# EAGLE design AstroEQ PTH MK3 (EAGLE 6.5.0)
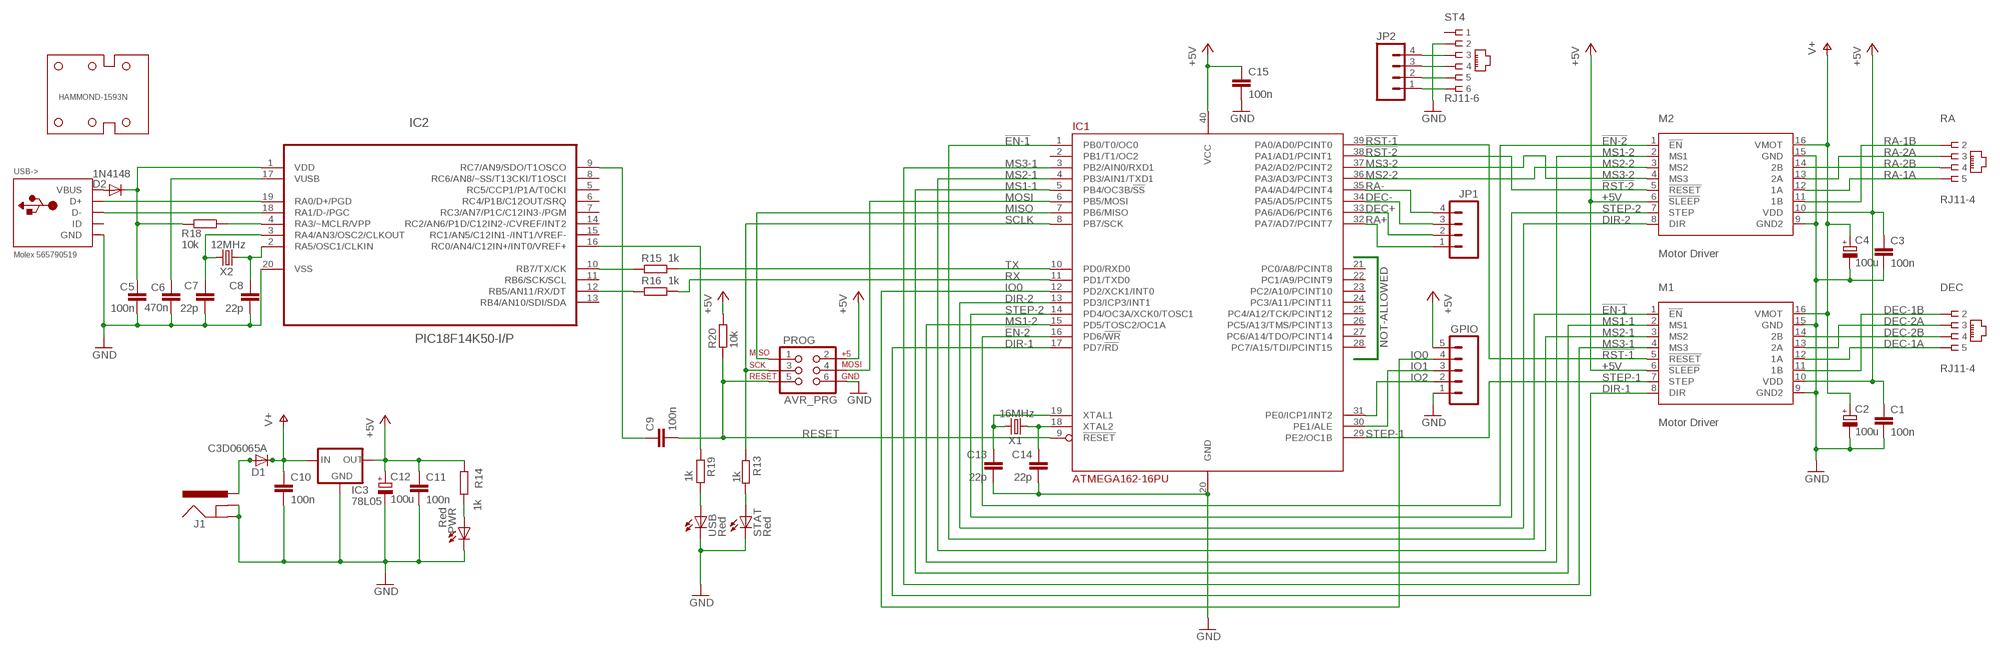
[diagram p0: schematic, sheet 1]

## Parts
C1  100n  C-EU025-024X044  [C025-024X044]
C2  100u  CPOL-EUE2.5-7  [E2,5-7]
C3  100n  C-EU025-024X044  [C025-024X044]
C4  100u  CPOL-EUE2.5-7  [E2,5-7]
C5  100n  C-EU025-024X044  [C025-024X044]
C6  470n  C-EU025-024X044  [C025-024X044]
C7  22p  C-EU025-024X044  [C025-024X044]
C8  22p  C-EU025-024X044  [C025-024X044]
C9  100n  C-EU025-024X044  [C025-024X044]
C10  100n  C-EU025-024X044  [C025-024X044]
C11  100n  C-EU025-024X044  [C025-024X044]
C12  100u  CPOL-EUE2.5-7  [E2,5-7]
C13  22p  C-EU025-024X044  [C025-024X044]
C14  22p  C-EU025-024X044  [C025-024X044]
C15  100n  C-EU025-024X044  [C025-024X044]
D1  C3D06065A  MUR820  [C221B1A]
D2  1N4148  DIODE1N4148  [DIODE-1N4148]
DEC  RJ11-4  [RJ11-NO_SHIELD-4]
GPIO  M05PTH  [1X05]
HAMMOND-1593N  HAMMOND-1593N  [HAMMOND-1593N]
IC1  ATMEGA162-16PU  [DIL40]
IC2  PIC18F14K50-I/P  [DIL20]
IC3  78L05  V_REG_78XXTO-92  [TO-92]
J1  POWER_JACKPTH  [POWER_JACK_PTH]
JP1  M04PTH  [1X04]
JP2  M04PTH  [1X04]
M1  Motor Driver  A4983CARRIER  [DIP16-W]
M2  Motor Driver  A4983CARRIER  [DIP16-W]
PROG  AVR_PRG  AVR_SPI_PRG_6PTH  [2X3]
PWR  Red  LED3MM  [LED3MM]
R13  1k  R-EU_0204/7  [0204/7]
R14  1k  R-EU_0204/7  [0204/7]
R15  1k  R-EU_0204/7  [0204/7]
R16  1k  R-EU_0204/7  [0204/7]
R18  10k  R-EU_0204/7  [0204/7]
R19  1k  R-EU_0204/7  [0204/7]
R20  10k  R-EU_0204/7  [0204/7]
RA  RJ11-4  [RJ11-NO_SHIELD-4]
ST4  RJ11-6  RJ11-2L-B  [RJ11-NO_SHIELD]
STAT  Red  LED3MM  [LED3MM]
USB  Red  LED3MM  [LED3MM]
USB->  Molex 565790519  USBMOLEX  [USB-MINIB-THM-MOLEX]
X1  16MHz  CRYSTALHC49US  [HC49US]
X2  12MHz  CRYSTALHC49US  [HC49US]

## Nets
!EN-1: IC1.1(PB0/T0/OC0) M1.1(!EN)
!EN-2: IC1.16(PD6/!WR) M2.1(!EN)
!RST-1: IC1.39(PA0/AD0/PCINT0) M1.5(!RESET)
!RST-2: IC1.38(PA1/AD1/PCINT1) M2.5(!RESET)
+5V: C1.1 C3.1 C11.1 C12.+ C15.1 GPIO.5 IC1.40(VCC) IC3.1(OUT) M1.6(!SLEEP) M1.10(VDD) M2.6(!SLEEP) M2.10(VDD) PROG.2 R14.1 R20.2
AVROSC1: C13.1 IC1.19(XTAL1) X1.2
AVROSC2: C14.1 IC1.18(XTAL2) X1.1
D+: IC2.19(RA0/D+/PGD) USB->.D+
D-: IC2.18(RA1/D-/PGC) USB->.D-
DEC+: IC1.33(PA6/AD6/PCINT6) JP1.2
DEC+B: JP2.2 ST4.5
DEC-: IC1.34(PA5/AD5/PCINT5) JP1.3
DEC-1A: DEC.5 M1.12(1A)
DEC-1B: DEC.2 M1.11(1B)
DEC-2A: DEC.3 M1.13(2A)
DEC-2B: DEC.4 M1.14(2B)
DEC-B: JP2.3 ST4.4
DIR-1: IC1.17(PD7/!RD) M1.8(DIR)
DIR-2: IC1.13(PD3/ICP3/INT1) M2.8(DIR)
DTR: C9.1 IC2.9(RC7/AN9/SDO/T1OSCO)
GND: C1.2 C2.- C3.2 C4.- C5.2 C6.1 C7.2 C8.2 C10.2 C11.2 C12.- C13.2 C14.2 C15.2 GPIO.1 IC1.20(GND) IC2.20(VSS) IC3.2(GND) J1.GND J1.GNDBREAK M1.9(GND2) M1.15(GND) M2.9(GND2) M2.15(GND) PROG.6 PWR.K(C) ST4.2 STAT.K(C) USB->.GND USB->.GND1(GND) USB->.GND4(GND) USB.K(C)
IO0: GPIO.4 IC1.12(PD2/XCK1/INT0)
IO1: GPIO.3 IC1.30(PE1/ALE)
IO2: GPIO.2 IC1.31(PE0/ICP1/INT2)
MCLR: IC2.4(RA3/~MCLR/VPP) R18.1
MISO: IC1.7(PB6/MISO) PROG.1
MOSI: IC1.6(PB5/MOSI) PROG.4
MS1-1: IC1.5(PB4/OC3B/!SS) M1.2(MS1)
MS1-2: IC1.15(PD5/TOSC2/OC1A) M2.2(MS1)
MS2-1: IC1.4(PB3/AIN1/TXD1) M1.3(MS2)
MS2-2: IC1.36(PA3/AD3/PCINT3) M2.3(MS2)
MS3-1: IC1.3(PB2/AIN0/RXD1) M1.4(MS3)
MS3-2: IC1.37(PA2/AD2/PCINT2) M2.4(MS3)
PWRLED: PWR.A R14.2
RA+: IC1.32(PA7/AD7/PCINT7) JP1.1
RA+B: JP2.1 ST4.6
RA-: IC1.35(PA4/AD4/PCINT4) JP1.4
RA-1A: M2.12(1A) RA.5
RA-1B: M2.11(1B) RA.2
RA-2A: M2.13(2A) RA.3
RA-2B: M2.14(2B) RA.4
RA-B: JP2.4 ST4.3
RESET: C9.2 IC1.9(!RESET) PROG.5 R20.1
RX: IC1.11(PD1/TXD0) R16.1
RX(USB): IC2.12(RB5/AN11/RX/DT) R16.2
SCLK: IC1.8(PB7/SCK) PROG.3 R13.1
STATLED: R13.2 STAT.A
STEP-1: IC1.29(PE2/OC1B) M1.7(STEP)
STEP-2: IC1.14(PD4/OC3A/XCK0/TOSC1) M2.7(STEP)
TX: IC1.10(PD0/RXD0) R15.1
TX(USB): IC2.10(RB7/TX/CK) R15.2
USBLED: R19.1 USB.A
USBOSC1: C8.1 IC2.2(RA5/OSC1/CLKIN) X2.1
USBOSC2: C7.1 IC2.3(RA4/AN3/OSC2/CLKOUT) X2.2
USBSTAT: IC2.16(RC0/AN4/C12IN+/INT0/VREF+) R19.2
V+: C2.+ C4.+ C10.1 D1.C IC3.3(IN) M1.16(VMOT) M2.16(VMOT)
VBUS: D2.A USB->.VBUS
VIN: D1.A J1.PWR
VPIC: C5.1 D2.C IC2.1(VDD) R18.2
VUSB: C6.2 IC2.17(VUSB)
Unconnected: IC1.2(PB1/T1/OC2) IC1.21(PC0/A8/PCINT8) IC1.22(PC1/A9/PCINT9) IC1.23(PC2/A10/PCINT10) IC1.24(PC3/A11/PCINT11) IC1.25(PC4/A12/TCK/PCINT12) IC1.26(PC5/A13/TMS/PCINT13) IC1.27(PC6/A14/TDO/PCINT14) IC1.28(PC7/A15/TDI/PCINT15) IC2.5(RC5/CCP1/P1A/T0CKI) IC2.6(RC4/P1B/C12OUT/SRQ) IC2.7(RC3/AN7/P1C/C12IN3-/PGM) IC2.8(RC6/AN8/~SS/T13CKI/T1OSCI) IC2.11(RB6/SCK/SCL) IC2.13(RB4/AN10/SDI/SDA) IC2.14(RC2/AN6/P1D/C12IN2-/CVREF/INT2) IC2.15(RC1/AN5/C12IN1-/INT1/VREF-) ST4.1 USB->.ID

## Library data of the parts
C1 C3 C5 C9-C11 C15 = resistor:C-EU: CAPACITOR, European symbol; MF: AVX; MPN: SR205C104KAR; OC_FARNELL: 1100367
C2 C4 C12 = resistor:CPOL-EU: POLARIZED CAPACITOR, European symbol; MF: MULTICOMP; MPN: MCGPR25V107M6.3X11; OC_FARNELL: 9451188
C6 = resistor:C-EU: CAPACITOR, European symbol; MF: KEMET; MPN: C320C474M5U5TA; OC_FARNELL: 1457660
C7 C8 C13 C14 = resistor:C-EU: CAPACITOR, European symbol; MF: AVX; MPN: SR151A220JAR; OC_FARNELL: 1100369
D1 = diode:MUR820: DIODE; MF: CREE; MPN: C3D06065A; OC_FARNELL: 1864928
D2 = SparkFun:DIODE: Diode; MF: MULTICOMP; MPN: 1N4148.; OC_FARNELL: 9565124
DEC RA = con-tycoelectronics:RJ11-4; MF: MOLEX; MPN: 95501-2641; OC_FARNELL: 1560166
GPIO = SparkFun:M05: Header 5 Standard 5-pin 0.1" header. Use with straight break away headers (SKU : PRT-00116), right angle break away headers (PRT-00553), swiss pins (PRT-00743), machine pins (PRT-00117), and female headers (PRT-00115). Molex polarized connector foot print use with SKU : PRT-08230 with associated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
HAMMOND-1593N = holes:HAMMOND-1593N; MF: HAMMOND; MPN: 1593NBK; OC_FARNELL: 9287566
IC1 = atmel:ATMEGA162: 8-bit RISC MICROCONTROLLER 16K Bytes internal flash program memory 1K Bytes internal SRAM Upto 64K Bytes optional external memory space 512 Bytes EEPROM Two 8-bit timers Two 16-bit timers Dual programmable serial USARTs Master/Slave serial SPI interface Source: ATMEGA162_DIP40.lbr; MF: ATMEL; MPN: ATMEGA162-16PU; OC_FARNELL: 9171169
IC2 = microchip:PIC18F14K50-I/P: USB Flash Microcontrollers; MF: MICROCHIP; MPN: PIC18F14K50-I/P; OC_FARNELL: 1648501; OC_NEWARK: 77M3103; PACKAGE: DIP-20; SUPPLIER: Microchip
IC3 = SparkFun:V_REG_78XX: Voltage Regulator Standard 7805 5V regulator. IGO (Input Ground Output). Spark Fun Electronics SKU : COM-00107; MF: FAIRCHILD SEMICONDUCTOR; MPN: LM78L05ACZX; OC_FARNELL: 1467367
J1 = SparkFun:POWER_JACK: Power Jack This is the standard 5.5mm barrel jack for power. The PTH is the most common, proven, reliable, footprint. All others are experimental. The Slot footprint only works if the mill layer is transmitted to the PCB fab house so be warned. Spark Fun Electronics SKU : PRT-00119. Mating wall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; MF: MULTICOMP; MPN: MJ-179PH; OC_FARNELL: 1737246
JP1 JP2 = SparkFun:M04: Header 4 Standard 4-pin 0.1" header. Use with straight break away headers (SKU : PRT-00116), right angle break away headers (PRT-00553), swiss pins (PRT-00743), machine pins (PRT-00117), and female headers (PRT-00115). Molex polarized connector foot print use with SKU : PRT-08231 with associated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
M1 M2 = A4983Carrier:A4983CARRIER; MF: SAMTEC; MPN: CES-116-01-T-S; OC_FARNELL: 1667522
PROG = SparkFun:AVR_SPI_PRG_6: AVR ISP 6 Pin This is the reduced ISP connector for AVR programming. Common on Arduino. This footprint will take up less PCB space and can be used with a 10-pin to 6-pin adapter such as SKU: BOB-08508; MF: TE CONNECTIVITY / AMP; MPN: 826632-3; OC_FARNELL: 3418492
PWR STAT USB = led:LED: LED; MF: KINGBRIGHT; MPN: L-424HDT; OC_FARNELL: 1142499
R13-R16 R19 = rcl:R-EU_: RESISTOR, European symbol; MF: MULTICOMP; MPN: MF12 1K; OC_FARNELL: 9342400
R18 R20 = rcl:R-EU_: RESISTOR, European symbol; MF: MULTICOMP; MPN: MF12 10K; OC_FARNELL: 9342419
ST4 = con-tycoelectronics:RJ11: CORCOM Modular RJ Jacks No Shield Source: www.tycoelectronics.com .. ENG_DS_1654001_1099_RJ_L_0507.pdf; MF: TYCO ELECTRONICS; MPN: RJ11-2L-B; OC_FARNELL: unknown; OC_NEWARK: 83F4463
USB-> = adafruit:USB: USB Connectors USBMINIB - Surface Mount Female Mini-B USB Connector 4UConnector: 06564 By microbuilder.eu Thru-hole RA Female Mini-B USB Connector 4UConnector: 18732 By ladyada.net; MF: MOLEX; MPN: 565790519; OC_FARNELL: 1125347
X1 = SparkFun:CRYSTAL: Crystals; MF: TXC; MPN: 9B-16.000MEEJ-B; OC_FARNELL: 1842217
X2 = SparkFun:CRYSTAL: Crystals; MF: TXC; MPN: 9B-12.000MAAJ-B; OC_FARNELL: 1842203

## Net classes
1 power: width 0.61 mm, drill 0.711 mm, clearance 0.203 mm
2 gnd: width 0.305 mm, drill 0.711 mm, clearance 0.203 mm
3 usbvcc: width 0.508 mm, drill 0.711 mm, clearance 0.203 mm

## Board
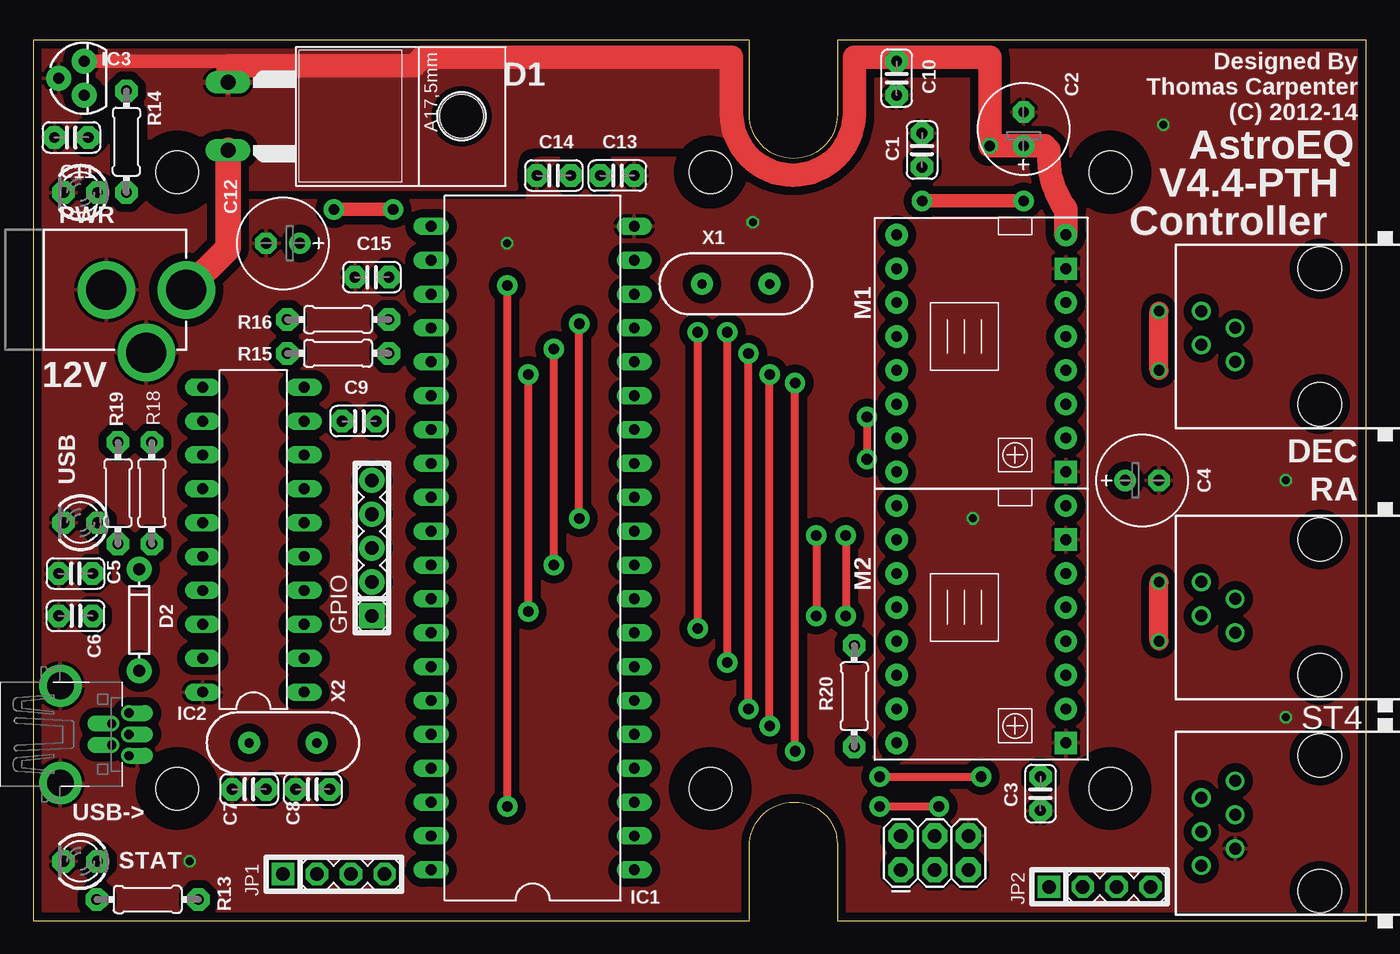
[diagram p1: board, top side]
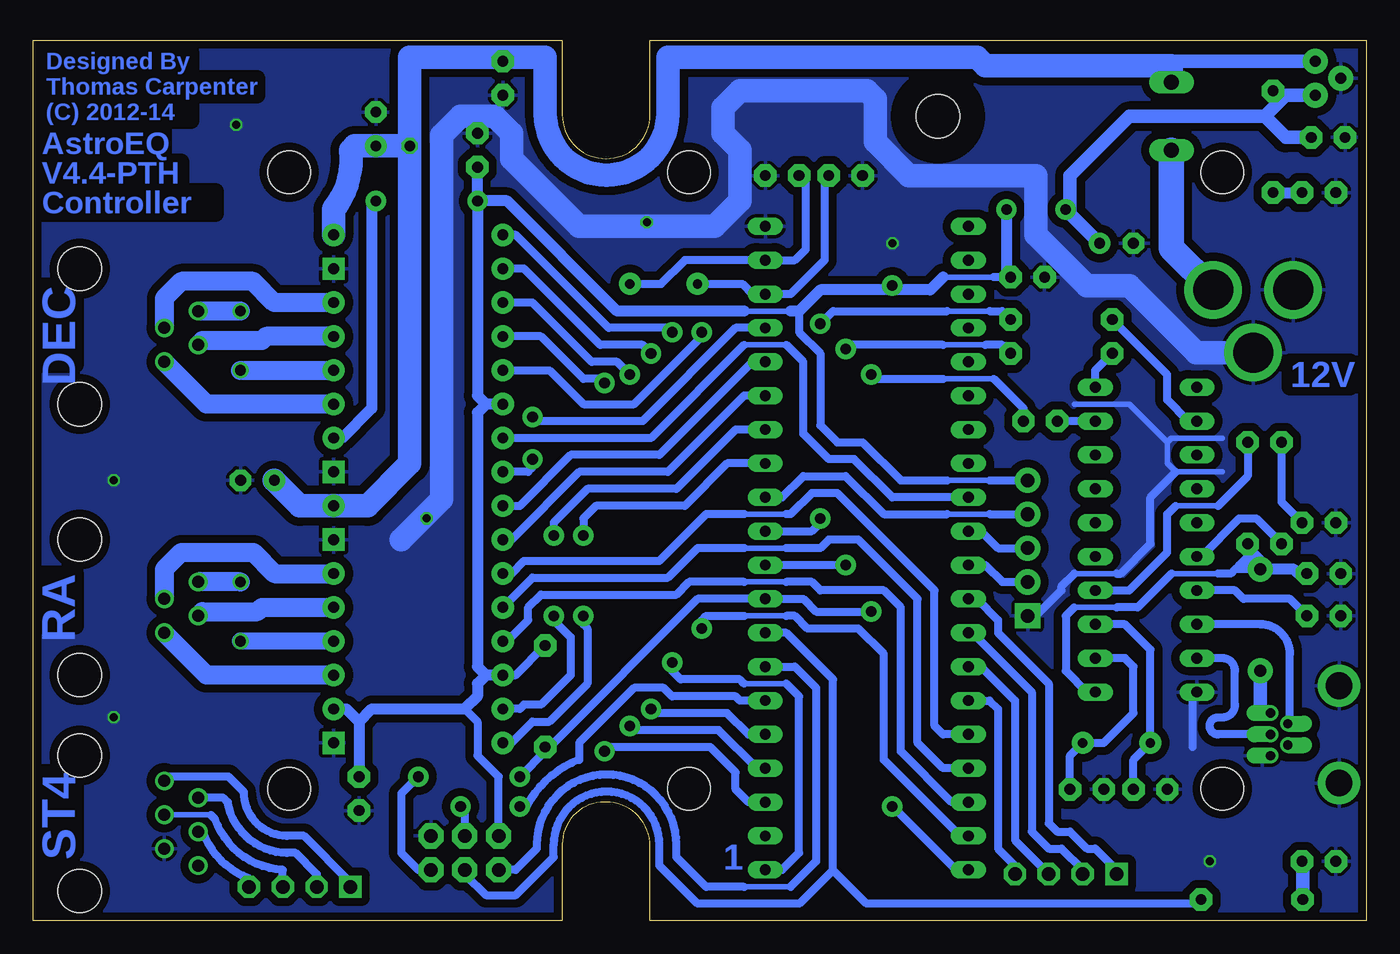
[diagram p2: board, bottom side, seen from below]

Size 100 x 66.04 mm. Coordinates in mm from the lower left corner, seen from the top.
Outline: 57.02,8.89 57.15,8.89
Copper layers (1*16): Top 0.035mm / dielectric 1.5mm / Bottom 0.035mm
Design rules "default *": minimum track width 6mil, minimum drill 12mil, track to track 6mil, track to pad 6mil, pad to pad 6mil, via to via 6mil, smd to smd 0mil, copper to edge 10mil, drill to drill 10mil, minimum pad ring 10mil, minimum via ring 6mil, stop-mask expansion 2mil, vias tented up to drill 1mm, thermal gap 10mil
tKeepout: area 78.3,7.4 to 83.3,12.4; area 78.3,53.6 to 83.3,58.6; area 48.3,7.4 to 53.3,12.4; area 8.3,7.4 to 13.3,12.4; area 48.3,53.6 to 53.3,58.6; area 8.3,53.6 to 13.3,58.6
bKeepout: area 78.3,7.4 to 83.3,12.4; area 78.3,53.6 to 83.3,58.6; area 48.3,7.4 to 53.3,12.4; area 8.3,7.4 to 13.3,12.4; area 48.3,53.6 to 53.3,58.6; area 8.3,53.6 to 13.3,58.6
tRestrict: area 78.3,53.6 to 83.3,58.6; area 78.3,7.4 to 83.3,12.4; area 48.3,7.4 to 53.3,12.4; area 8.3,7.4 to 13.3,12.4; area 8.3,53.6 to 13.3,58.6; area 6.3,56.2 to 7.9,60.6; 1 lines

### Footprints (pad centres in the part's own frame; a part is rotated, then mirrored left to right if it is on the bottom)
C025-024X044 = drill 0.813 pad 1.676 octagon: 1 -1.27,0; 2 1.27,0
E2,5-7 = drill 0.813 pad 1.6: + -1.27,0 | drill 0.813 pad 1.6 octagon: - 1.27,0
C221B1A = drill 1.118 long: A 2.54,-6.35; C -2.54,-6.35 | hole 3.302: 0,11.176
DIODE-1N4148 = drill 0.9 pad 1.88: A -3.81,0; C 3.81,0
RJ11-NO_SHIELD-4 = drill 0.9 pad 1.4: 2 -1.905,6.35; 3 -0.635,8.89; 4 0.635,6.35; 5 1.905,8.89 | hole 3.251: -5.08,0; 5.08,0
1X05 = drill 1.016 pad 1.88 square: 1 0,0 | drill 1.016 pad 1.88: 2 2.54,0; 3 5.08,0; 4 7.62,0; 5 10.16,0
HAMMOND-1593N = hole 3.2: 10.795,9.906; 10.795,56.134; 50.8,9.906; 50.8,56.134; 80.797,9.906; 80.797,56.134
DIL40 = drill 0.813 long: 1 -24.13,-7.62; 2 -21.59,-7.62; 3 -19.05,-7.62; 4 -16.51,-7.62; 5 -13.97,-7.62; 6 -11.43,-7.62; 7 -8.89,-7.62; 8 -6.35,-7.62; 9 -3.81,-7.62; 10 -1.27,-7.62; 11 1.27,-7.62; 12 3.81,-7.62; 13 6.35,-7.62; 14 8.89,-7.62; 15 11.43,-7.62; 16 13.97,-7.62; 17 16.51,-7.62; 18 19.05,-7.62; 19 21.59,-7.62; 20 24.13,-7.62; 21 24.13,7.62; 22 21.59,7.62; 23 19.05,7.62; 24 16.51,7.62; 25 13.97,7.62; 26 11.43,7.62; 27 8.89,7.62; 28 6.35,7.62; 29 3.81,7.62; 30 1.27,7.62; 31 -1.27,7.62; 32 -3.81,7.62; 33 -6.35,7.62; 34 -8.89,7.62; 35 -11.43,7.62; 36 -13.97,7.62; 37 -16.51,7.62; 38 -19.05,7.62; 39 -21.59,7.62; 40 -24.13,7.62
DIL20 = drill 0.813 long: 1 -3.81,11.43; 2 -3.81,8.89; 3 -3.81,6.35; 4 -3.81,3.81; 5 -3.81,1.27; 6 -3.81,-1.27; 7 -3.81,-3.81; 8 -3.81,-6.35; 9 -3.81,-8.89; 10 -3.81,-11.43; 11 3.81,-11.43; 12 3.81,-8.89; 13 3.81,-6.35; 14 3.81,-3.81; 15 3.81,-1.27; 16 3.81,1.27; 17 3.81,3.81; 18 3.81,6.35; 19 3.81,8.89; 20 3.81,11.43
TO-92 = drill 0.813 pad 1.88: 1 -1.27,0; 2 0,1.905; 3 1.27,0
POWER_JACK_PTH = drill 2.997 pad 4.318: GND 0,7.7; GNDBREAK 4.7,10.7; PWR 0,13.7
1X04 = drill 1.016 pad 1.676 square: 1 0,0 | drill 1.016 pad 1.676 octagon: 2 2.54,0; 3 5.08,0; 4 7.62,0
DIP16-W = drill 0.813 pad 1.676: 1 -8.89,-6.35; 2 -6.35,-6.35; 3 -3.81,-6.35; 4 -1.27,-6.35; 5 1.27,-6.35; 6 3.81,-6.35; 7 6.35,-6.35; 8 8.89,-6.35; 10 6.35,6.35; 11 3.81,6.35; 12 1.27,6.35; 13 -1.27,6.35; 14 -3.81,6.35; 16 -8.89,6.35 | drill 0.813 pad 1.676 square: 9 8.89,6.35; 15 -6.35,6.35
2X3 = drill 1.016 pad 1.88 octagon: 1 0,0; 2 0,2.54; 3 2.54,0; 4 2.54,2.54; 5 5.08,0; 6 5.08,2.54
LED3MM = drill 0.813 pad 1.676 octagon: A -1.27,0; K 1.27,0
0204/7 = drill 0.813 pad 1.676 octagon: 1 -3.81,0; 2 3.81,0
RJ11-NO_SHIELD = drill 0.9 pad 1.4: 1 -3.175,8.89; 2 -1.905,6.35; 3 -0.635,8.89; 4 0.635,6.35; 5 1.905,8.89; 6 3.175,6.35 | hole 3.251: -5.08,0; 5.08,0
USB-MINIB-THM-MOLEX = drill 0.7 offset: D+ 0,9.72; D- -0.8,8.42; GND 1.6,9.72; ID 0.8,8.42; VBUS -1.6,9.72 | drill 2 pad 3.175: GND1 -3.65,4.57; GND4 3.65,4.57
HC49US = drill 0.7 pad 1.651: 1 -2.54,0; 2 2.54,0

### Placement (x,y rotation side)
C1  66.67,57.78 90 top
C2  74.3,59.37 90 top
C3  75.56,9.53 270 top
C4  83.19,33.02 0 top
C5  3.17,26.04 180 top
C6  3.17,22.86 0 top
C7  16.19,9.84 180 top
C8  20.95,9.84 180 top
C9  24.45,37.47 0 top
C10  64.77,63.18 270 top
C11  2.86,58.74 180 top
C12  18.73,50.8 180 top
C13  43.81,55.88 0 top
C14  39.05,55.88 180 top
C15  25.4,48.26 180 top
D1  20.95,60.33 270 top
D2  7.94,22.54 90 top
DEC  96.52,43.81 90 top
GPIO  25.4,22.86 90 top
HAMMOND-1593N  0,0 0 top
IC1  37.47,27.94 90 top
IC2  16.51,28.57 180 top
IC3  3.81,63.18 90 top
J1  -2.22,47.31 270 top
JP1  18.73,3.49 0 top
JP2  76.2,2.54 0 top
M1  71.12,42.55 270 top
M2  71.12,22.23 270 top
PROG  65.09,3.81 0 top
PWR  3.54,54.61 180 top
R13  8.57,1.59 180 top
R14  6.99,58.42 270 top
R15  22.86,42.55 180 top
R16  22.86,45.09 180 top
R18  8.89,32.07 270 top
R19  6.35,32.07 270 top
R20  61.59,16.83 90 top
RA  96.52,23.5 90 top
ST4  96.52,7.3 90 top
STAT  3.54,4.45 180 top
USB  3.54,29.84 180 top
USB->  -2.54,13.97 270 top
X1  52.7,47.75 0 top
X2  18.73,13.34 180 top

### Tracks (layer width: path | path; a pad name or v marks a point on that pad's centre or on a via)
!EN-1  (via drill 0.8 pad 1.52)
  Top 0.61: v52.07,19.37 v52.07,44.13
  Bottom 0.406: 43.5,17.78 46.67,17.78
  Bottom 0.61: IC1.1 43.81,3.81 42.55,5.08 42.55,16.83 43.5,17.78 | 46.67,17.78 46.99,18.1 51.44,18.1 52.07,18.73 v52.07,19.37 | v52.07,44.13 52.39,44.45 56.83,44.45 63.82,51.44 M1.1
!EN-2
  Bottom 0.61: IC1.16 46.04,41.91 53.02,34.92 59.69,34.92 63.5,31.11 M2.1
!RST-1  (via drill 0.8 pad 1.52)
  Top 0.61: v49.85,44.13 v49.85,21.91
  Bottom 0.406: 43.5,22.86 46.67,22.86
  Bottom 0.61: IC1.39 30.48,6.35 36.2,12.06 36.2,20 38.1,21.91 41.91,21.91 42.86,22.86 43.5,22.86 | M1.5 61.28,41.27 58.74,38.73 54.93,38.73 49.85,43.81 v49.85,44.13 | v49.85,21.91 49.85,22.54 49.53,22.86 46.67,22.86
!RST-2
  Bottom 0.406: 43.5,25.4 46.67,25.4
  Bottom 0.61: IC1.38 31.11,8.89 34.92,12.7 34.92,23.5 36.2,24.77 40.96,24.77 41.59,25.4 43.5,25.4 | 46.67,25.4 50.8,25.4 51.75,24.45 61.91,24.45 62.87,23.5 62.87,22.54 64.45,20.95 M2.5
+5V  (via drill 0.8 pad 1.52)
  Top 0.61: v35.56,47.62 v35.56,8.57
  Top 1.016: v66.67,53.98 v74.3,53.98 | v22.54,53.34 v26.99,53.34
  Bottom 0.406: 27.94,48.26 31.75,48.26 | 43.18,45.72 46.67,45.72 | 31.43,33.02 28.26,33.02
  Bottom 0.61: 26.99,48.26 27.94,48.26 | PROG.2 65.09,10.79 66.67,12.38 66.67,14.92 67.63,15.88 | v35.56,47.62 35.56,47.31 | IC1.40 30.8,3.81 v35.56,8.57 | M2.6 63.82,18.41 R20.2 | 42.55,45.72 42.55,44.13 40.96,42.55 40.96,37.15 39.69,35.88 37.78,35.88 34.92,33.02 31.43,33.02 | 28.26,33.02 GPIO.5
  Bottom 0.813: v66.67,53.98 C1.1 | C15.1 26.99,48.26 v26.99,53.34 | 31.75,48.26 32.7,47.31 35.56,47.31 40.96,47.31 42.55,45.72 43.18,45.72 | 46.67,45.72 56.2,45.72 64.45,53.98 v66.67,53.98 | 22.23,53.66 22.23,53.34 v22.54,53.34 | v66.67,53.98 66.67,39.37 66.04,38.73 | 66.04,38.73 66.67,38.1 66.67,19.05 66.04,18.41 | 66.04,18.41 66.67,17.78 66.67,16.83 67.63,15.88 74.61,15.88 75.56,14.92 | M2.6 66.04,18.41 | M1.6 66.04,38.73 | v74.3,53.98 74.61,53.66 74.61,38.42 76.83,36.2 M1.10 | 75.56,14.92 C3.1 | M2.10 76.52,15.88 75.56,14.92
  Bottom 1.016: IC3.1 6.03,61.91 6.35,61.59 | 6.35,61.59 7.62,60.33 | 7.62,60.33 17.78,60.33 22.23,55.88 22.23,53.66 22.23,53.02 C12.+ | R14.1 6.35,61.59 | C11.1 6.03,58.74 7.62,60.33
AVROSC1
  Bottom 0.61: C13.1 42.07,55.4 42.07,50.32 42.86,49.53 IC1.19 51.12,49.53 52.9,47.75 X1.2
AVROSC2
  Bottom 0.61: C14.1 40.64,55.56 40.64,49.53 43.18,46.99 IC1.18 46.04,46.99 46.8,47.75 X1.1
D+
  Bottom 0.61: USB->.D+ 11.11,13.97 arc90 11.75,14.61 arc90 11.11,15.24 10.79,15.24 arc-90 9.84,16.19 9.84,18.73 arc-90 10.79,19.68 IC2.19
D-
  Bottom 0.61: USB->.D- 5.71,14.77 5.71,20 arc-90 7.94,22.23 IC2.18
DEC+
  Bottom 0.61: IC1.33 29.53,21.59 25.08,17.14 25.08,6.67 23.81,5.4 22.86,5.4 21.27,3.81 JP1.2
DEC+B
  Bottom 0.61: JP2.2 78.74,3.49 80.33,5.08 80.96,5.08 arc80 85.41,8.89 85.72,9.21 ST4.5
DEC-
  Bottom 0.61: IC1.34 28.89,19.05 26.35,16.51 26.35,6.03 JP1.3
DEC-1A  (via drill 0.8)
  Top 1.422: v84.45,41.27 v84.45,45.72
  Bottom 1.422: v84.45,45.72 DEC.5 | v84.45,41.27 M1.12
DEC-1B
  Bottom 1.422: M1.11 87,38.73 DEC.2
DEC-2A
  Bottom 1.422: M1.13 82.55,43.81 82.87,43.5 87.31,43.5 DEC.3
DEC-2B
  Bottom 1.422: M1.14 81.92,46.35 83.5,47.94 88.9,47.94 90.17,46.67 DEC.4
DEC-B
  Bottom 0.406: 86.68,7.94 ST4.4
  Bottom 0.61: 86.68,7.94 86.36,7.62 arc-68 81.28,3.81 JP2.3
DIR-1  (via drill 0.8 pad 1.52)
  Top 0.61: v62.55,37.78 v62.55,34.61
  Bottom 0.61: IC1.17 47.31,44.45 54.29,37.47 62.23,37.47 v62.55,37.78 | v62.55,34.61 62.55,33.97 62.87,33.66 M1.8
DIR-2  (via drill 0.8 pad 1.52)
  Top 0.61: v58.74,28.89 v58.74,22.86
  Bottom 0.61: M2.8 64.14,13.34 62.55,14.92 61.28,14.92 58.42,17.78 58.42,21.91 58.74,22.23 v58.74,22.86 | IC1.13 47.94,34.29 51.12,31.11 57.78,31.11 58.74,30.16 v58.74,28.89
DTR
  Bottom 0.61: IC2.9 C9.1
GND  (via drill 0.6)
  Bottom 0.406: 21.91,26.04 18.73,26.04 | 10.79,33.66 14.29,33.66 14.92,34.29 14.92,35.88 | 14.92,35.88 14.61,36.2 10.79,36.2 | 14.92,35.88 17.78,38.73 21.91,38.73
  Bottom 0.61: 13.02,13.02 13.02,16.83 IC2.20 | GPIO.1 24.77,22.86 22.86,24.77 22.86,25.08 21.91,26.04 | 18.73,26.04 18.41,26.04 16.19,28.26 16.19,31.75 14.29,33.66
  Bottom 1.778: J1.GNDBREAK 12.76,42.61 17.78,47.62 20.95,47.62 24.77,51.44 24.77,55.88 34.29,55.88 36.83,58.42 36.83,61.59 37.47,62.23 46.99,62.23 48.26,60.96 48.26,59.05 46.99,57.78 46.99,53.98 48.9,52.07 59.05,52.07 64.14,57.15 64.14,59.05 65.41,60.33 67.94,60.33 69.37,58.9 69.37,31.59 72.39,28.57
  other vias: 35.56,50.8 93.98,15.24 84.77,59.69 93.98,33.02 70.48,30.16 53.98,52.39 11.75,4.45
  pour Top (isolate 0.61, rank 2): -1.27,66.99 101.03,66.99 101.03,-0.95 -1.27,-0.95
  pour Bottom (isolate 0.61): -1.27,66.99 101.03,66.99 101.03,-0.95 -1.27,-0.95
IO0
  Bottom 0.406: 31.43,30.48 28.26,30.48
  Bottom 0.61: IC1.12 43.81,31.75 42.23,33.34 39.05,33.34 36.2,30.48 31.43,30.48 | 28.26,30.48 GPIO.4
IO1
  Bottom 0.61: IC1.30 28.89,29.21 27.62,27.94 GPIO.3
IO2
  Bottom 0.61: IC1.31 28.57,26.67 27.3,25.4 GPIO.2
MCLR
  Bottom 0.406: 14.29,31.11 11.11,31.11
  Bottom 0.61: IC2.4 17.78,24.77 14.92,27.62 14.92,30.48 14.29,31.11 | 11.11,31.11 8.89,33.34 R18.1
MISO
  Bottom 0.406: 43.18,2.54 46.67,2.54
  Bottom 0.61: IC1.7 42.86,19.05 41.27,17.46 41.27,4.45 43.18,2.54 | 46.67,2.54 49.53,2.54 51.75,4.76 51.75,5.71 arc-180 62.23,5.71 62.23,5.4 63.82,3.81 PROG.1
MOSI  (via drill 0.8 pad 1.52)
  Top 0.61: v63.5,8.57 v67.94,8.57
  Bottom 0.61: IC1.6 46.99,16.51 47.31,16.83 52.07,16.83 52.7,17.46 54.93,17.46 59.05,13.34 59.05,12.06 arc-42 63.01,8.57 v63.5,8.57 | v67.94,8.57 67.63,8.26 PROG.4
MS1-1  (via drill 0.8 pad 1.52)
  Top 0.61: v53.66,15.88 v53.66,42.55
  Bottom 0.61: IC1.5 46.35,13.97 47.94,15.56 53.34,15.56 v53.66,15.88 | v53.66,42.55 54.29,43.18 57.47,43.18 63.18,48.9 M1.2
MS1-2
  Bottom 0.61: IC1.15 46.67,39.37 52.39,33.66 59.05,33.66 64.14,28.57 M2.2
MS2-1  (via drill 0.8 pad 1.52)
  Top 0.61: v55.24,14.61 v55.24,40.96
  Bottom 0.61: IC1.4 45.72,11.43 48.58,14.29 54.93,14.29 v55.24,14.61 | v55.24,40.96 56.2,41.91 58.1,41.91 62.55,46.35 M1.3
MS2-2
  Bottom 0.406: 43.5,30.48 46.67,30.48
  Bottom 0.61: IC1.36 31.75,13.97 32.38,14.61 32.38,24.77 39.69,32.07 41.59,32.07 43.18,30.48 43.5,30.48 | 46.67,30.48 49.53,30.48 53.02,26.99 63.18,26.99 64.14,26.04 M2.3
MS3-1  (via drill 0.8 pad 1.52)
  Top 0.61: v57.15,12.7 v57.15,40.32
  Bottom 0.61: IC1.3 46.35,8.89 47.31,9.84 47.31,11.11 49.21,13.02 56.83,13.02 v57.15,12.7 | v57.15,40.32 57.47,40.64 58.74,40.64 61.91,43.81 M1.4
MS3-2
  Bottom 0.406: 43.5,27.94 46.67,27.94
  Bottom 0.61: IC1.37 31.75,11.43 33.66,13.34 33.66,24.13 38.1,28.57 40.32,28.57 40.96,27.94 43.5,27.94 | 46.67,27.94 50.16,27.94 52.39,25.72 62.55,25.72 M2.4
PWRLED
  Bottom 0.813: R14.2 PWR.A
RA+
  Bottom 0.61: IC1.32 29.21,24.13 27.62,22.54 27.62,21.59 23.81,17.78 23.81,7.3 23.18,6.67 22.23,6.67 20.95,5.4 20.32,5.4 18.73,3.81 JP1.1
RA+B
  Bottom 0.61: JP2.1 76.2,2.86 79.69,6.35 80.96,6.35 arc90 84.2,9.65 85.34,10.79 89.85,10.79 ST4.6
RA-
  Bottom 0.61: IC1.35 28.26,16.51 27.62,15.88 27.62,5.4 26.35,4.13 JP1.4
RA-1A  (via drill 0.8)
  Top 1.422: v84.45,20.95 v84.45,25.4
  Bottom 1.27: M2.12 v84.45,20.95
  Bottom 1.422: v84.45,25.4 RA.5
RA-1B
  Bottom 1.422: M2.11 87,18.41 RA.2
RA-2A
  Bottom 1.422: RA.3 87.31,23.18 83.19,23.18 82.87,23.5 M2.13
RA-2B
  Bottom 1.422: M2.14 81.92,26.04 83.5,27.62 88.9,27.62 90.17,26.35 RA.4
RA-B
  Bottom 0.61: ST4.3 87.31,6.67 arc-48 83.82,3.17 JP2.4
RESET  (via drill 0.8 pad 1.52)
  Top 0.61: v63.5,10.79 v71.12,10.79 | v37.15,23.18 v37.15,40.96
  Bottom 0.406: 31.75,40.64 27.94,40.64
  Bottom 0.61: v63.5,10.79 61.59,12.7 R20.1 61.28,13.02 50.16,24.13 IC1.9 42.23,24.13 41.27,23.18 v37.15,23.18 | v71.12,10.79 72.39,9.53 72.39,5.08 71.12,3.81 PROG.5 | v37.15,40.96 36.83,40.64 31.75,40.64 | 27.94,40.64 25.72,38.42 C9.2
RX  (via drill 0.8 pad 1.52)
  Top 0.61: v40.96,30.16 v40.96,44.77
  Bottom 0.406: 31.43,45.72 28.26,45.72
  Bottom 0.61: 31.43,45.72 40.01,45.72 v40.96,44.77 | 28.26,45.72 27.3,45.72 R16.1 | IC1.11 41.59,29.21 40.96,29.84 v40.96,30.16
RX(USB)
  Bottom 0.61: IC2.12 13.34,37.47 14.92,39.05 14.92,40.96 R16.2
SCLK
  Bottom 0.61: R13.1 12.7,1.27 37.49,1.27 40.01,3.79 | 40.01,3.79 40.01,18.1 43.5,21.59 IC1.8 | 40.01,3.79 42.52,1.27 50.16,1.27 53.02,4.13 53.02,5.71 arc-180 60.96,5.71 60.96,4.76 63.82,1.91 66.04,1.91 67.63,3.49 PROG.3
STATLED
  Bottom 1.016: STAT.A 4.76,4.49 R13.2
STEP-1
  Bottom 0.406: 43.5,43.18 46.67,43.18
  Bottom 0.61: IC1.29 35.56,31.75 38.42,34.61 40.32,34.61 42.23,36.51 42.23,41.91 43.5,43.18 | 46.67,43.18 53.66,36.2 M1.7
STEP-2  (via drill 0.8 pad 1.52)
  Top 0.61: v60.96,28.89 v60.96,22.86
  Bottom 0.61: IC1.14 47.31,36.83 51.75,32.38 58.42,32.38 60.96,29.84 v60.96,28.89 | v60.96,22.86 60.96,22.54 59.69,21.27 59.69,18.41 61.91,16.19 63.18,16.19 63.5,15.88 M2.7
TX  (via drill 0.8 pad 1.52)
  Top 0.61: v39.05,26.67 v39.05,42.86
  Bottom 0.406: 28.57,43.18 31.75,43.18
  Bottom 0.61: v39.05,26.67 IC1.10 | R15.1 27.3,43.18 28.57,43.18 | 31.75,43.18 38.73,43.18 v39.05,42.86
TX(USB)
  Bottom 0.61: IC2.10 20.32,41.27 R15.2
USBLED
  Bottom 0.61: USB.A 6.35,31.39 R19.1
USBOSC1
  Bottom 0.61: IC2.2 18.1,19.68 17.46,19.05 17.46,15.56 19.68,13.34 X2.1 22.23,12.38 C8.1
USBOSC2
  Bottom 0.61: IC2.3 18.1,22.23 16.19,20.32 X2.2 17.46,12.06 C7.1
USBSTAT
  Bottom 0.61: IC2.16 12.38,27.3 9.53,30.16 8.26,30.16 R19.2
V+  (via drill 0.8)
  Top 1.016: IC3.3 14.61,64.45 14.61,63.82
  Top 1.778: 14.61,63.82 D1.C 14.61,64.14 28.57,64.14 29.21,64.77 52.39,64.77 52.39,60.52 arc180 61.59,60.52 61.59,64.77 71.75,64.77 v71.75,58.1 C2.+ 75.88,58.1 76.2,57.78 76.2,57.15 arc37 77.47,53.34 M1.16
  Bottom 0.61: C10.1 64.77,64.77 | D1.C 14.61,63.5 14.61,64.45 14.29,64.45
  Bottom 1.016: IC3.3 14.29,64.45
  Bottom 1.778: v71.75,58.1 71.75,64.77 64.77,64.77 61.59,64.77 61.59,60.52 arc-180 52.39,60.52 52.39,64.77 29.21,64.77 28.57,64.14 14.61,64.14 14.61,63.5 | v71.75,58.1 C2.+ 75.88,58.1 76.2,57.78 arc45 77.47,53.34 M1.16 | v71.75,58.1 71.75,34.29 74.93,31.11 M2.16 80.01,31.11 C4.+
  pour Top (isolate 0.61): 3.17,66.04 3.17,61.28 6.99,61.28 6.99,54.93 36.2,54.93 36.2,56.83 arc-90 37.47,58.1 50.8,58.1 50.8,57.47 57.15,57.47 57.15,66.04
VBUS
  Bottom 1.016: USB->.VBUS 7.94,15.57 D2.A
VIN
  Top 1.93: J1.PWR 14.61,50.44 D1.A
  Bottom 1.93: J1.PWR 14.61,50.44 D1.A
VPIC
  Bottom 0.406: 11.11,26.04 14.61,26.04 | 18.73,23.5 21.91,23.5
  Bottom 0.61: 14.61,26.04 17.14,23.5 18.73,23.5 | 21.91,23.5 22.54,22.86 22.54,18.73 20.95,17.14 IC2.1 | 11.11,26.04 10.16,26.04 9.84,26.35 | D2.C 9.84,26.35 | 9.84,26.35 9.53,26.67 | 8.57,27.62 9.53,26.67 | 9.53,26.67 8.89,26.67 8.26,27.3
  Bottom 0.813: C5.1 5.08,26.04 5.4,26.35 D2.C 7.94,26.99 8.57,27.62 8.89,27.94 R18.2
VUSB
  Bottom 0.61: C6.2 5.71,24.13 9.21,24.13 9.84,24.77 IC2.17

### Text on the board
Bottom: Designed By | Thomas Carpenter | (C) 2012-14 | AstroEQ | V4.4-PTH | Controller | DEC | 12V | RA | ST4 | 1
tNames: Designed By | Thomas Carpenter | (C) 2012-14 | AstroEQ | V4.4-PTH | Controller | 12V
tValues: Sq Pad | 8824/5 | 4988 | 8824/5 | Sq Pad | 4988 | Markings show the location of the Potentiometers on the | Pololu Boards depending on which chip they use.
Reference: This board design is for DIY/Kit AstroEQ boards | It is a 2 Layer board designed to be sent for manufacture. The AstroEQ-PTH-Gerber.zip file contains the required gerber files. | I use iteadstudio.com 10cm x 10cm prototype service, selecting 1.2mm thick, HASL, 100% electrical check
